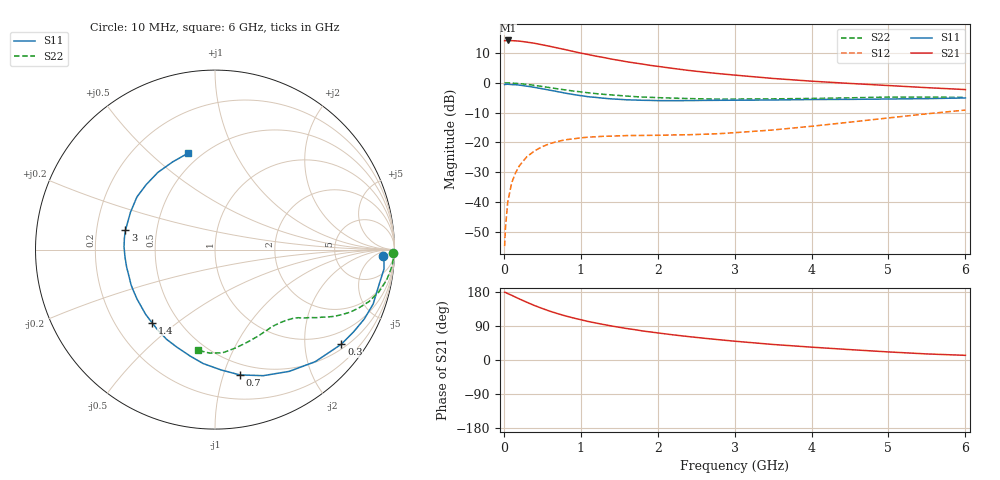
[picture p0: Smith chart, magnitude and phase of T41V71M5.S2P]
! Infineon Technologies  Discrete & RF Semiconductors
! BFR182T
! Si NPN RF Bipolar Junction Transistor in SC75
! VCE = 1.75 V  IC = 1.5 mA
! Common Emitter S-Parameters:  October  1999
# GHz  S  MA  R  50
!  f  S11  S21  S12  S22
! GHz  MAG  ANG  MAG  ANG  MAG  ANG  MAG  ANG
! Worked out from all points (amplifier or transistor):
!   36 points, 10 MHz to 6 GHz, reference 50 ohm
!   highest |S21| = 14.2 dB at 50 MHz (marker M1)
!   |S21| within 3 dB of that: start of sweep to 784.3 MHz
!   unconditionally stable (mu >= 1): 2.131 GHz to 4.512 GHz
!   at 250 MHz: K = 0.13, MSG = 20.1 dB, |S12| = -26.4 dB
!   at 1.4 GHz: K = 0.70, MSG = 12.9 dB, |S12| = -17.9 dB
!   at 6 GHz: K = 0.84, MSG = 3.4 dB, |S12| = -9.1 dB
!   S11 on the Smith chart (normalised r, x): 10 MHz: 22, -13; 300 MHz: 0.62, -2.89; 700 MHz: 0.40, -1.14; 1.4 GHz: 0.36, -0.41; 3 GHz: 0.33, +0.10; 6 GHz: 0.43, +0.67
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0.01  0.9348 -2.3  5.121 178.6  0.0018 82.2  0.9904 -1.2
0.02  0.9412 -1.2  5.115 178.5  0.0035 87.1  0.9999 -1.0
0.05  0.948 -6.5  5.156 175.3  0.0098 91.1  0.9953 -2.6
0.1  0.9344 -12.1  5.112 171.0  0.0205 85.4  0.991 -5.1
0.15  0.932 -19.0  5.084 166.0  0.0303 79.8  0.9812 -7.6
0.2  0.9173 -24.9  5.026 161.3  0.0401 76.6  0.9711 -10.0
0.3  0.8795 -36.8  4.829 152.3  0.0575 69.4  0.9428 -14.5
0.4  0.8381 -48.1  4.619 143.6  0.072 63.4  0.9061 -18.6
0.5  0.7947 -58.6  4.358 136.0  0.0847 58.4  0.868 -21.8
0.6  0.7519 -69.1  4.105 128.7  0.0954 53.9  0.8305 -24.8
0.7  0.7116 -78.8  3.85 122.3  0.1037 49.9  0.7934 -27.2
0.9  0.638 -96.0  3.378 111.1  0.1145 43.8  0.7293 -31.0
1.1  0.5839 -111.2  2.985 101.5  0.1223 39.7  0.6802 -33.9
1.4  0.5374 -130.9  2.506 89.8  0.1271 36.0  0.6268 -37.4
1.8  0.5093 -153.0  2.069 76.8  0.1306 35.0  0.5773 -41.7
2.2  0.5019 -168.8  1.747 66.4  0.1331 37.0  0.5538 -46.0
2.6  0.507 178.3  1.515 57.5  0.1368 40.7  0.5381 -51.2
3  0.5105 167.8  1.35 49.6  0.1454 45.1  0.5341 -56.1
3.5  0.515 156.0  1.185 41.0  0.1616 51.0  0.5383 -63.4
4.5  0.5274 136.5  0.977 27.4  0.2185 57.3  0.5602 -78.3
5.5  0.5427 115.7  0.83 16.0  0.3018 56.6  0.5771 -93.0
6  0.5575 105.7  0.771 12.3  0.3489 53.7  0.569 -99.8
